(* Logix 5000 AddOnInstructionDefinition export AMCI_SD4840E2_Jog_CCW; software revision 20.03 *)

ADD_ON_INSTRUCTION AMCI_SD4840E2_Jog_CCW   (* revision 1.0, vendor AMCI, ExecuteEnableInFalse *)
VAR_INPUT
   Axis_Status_Bits : INT; {required}
   Programmed_Speed : DINT; {required}
   Acceleration : INT; {required}
   Deceleration : INT; {required}
   Jerk : INT;
END_VAR
VAR_OUTPUT
   EN : BOOL; {access Read Only, visible}
   Jog_CCW_Occurring : BOOL; {access Read Only, visible}
END_VAR
VAR_IN_OUT
   AMCI_SD4840E2_output_data : _000A:SD4840E2_4342D302:O:0; {required}
END_VAR
VAR_OUTPUT
   ER : BOOL; {access Read Only, visible}
END_VAR
VAR
   Upper_Result_X_1000 : DINT;
   command_data_block : INT[10];
        [0]   // Command Bits MSW
        [1]   // Command Bits LSW
        [2]   // Upper Target Position
        [3]   // Lower Target Position
        [4]   // Upper Programmed Speed
        [5]   // Lower Programmed Speed
END_VAR

ROUTINE EnableInFalse   (* ladder *)
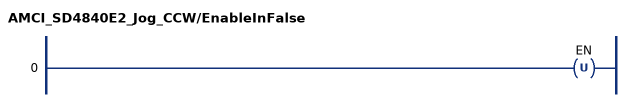
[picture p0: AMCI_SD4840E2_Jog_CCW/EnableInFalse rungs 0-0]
   0: OTU(EN);
END_ROUTINE

ROUTINE Logic   (* ladder *)
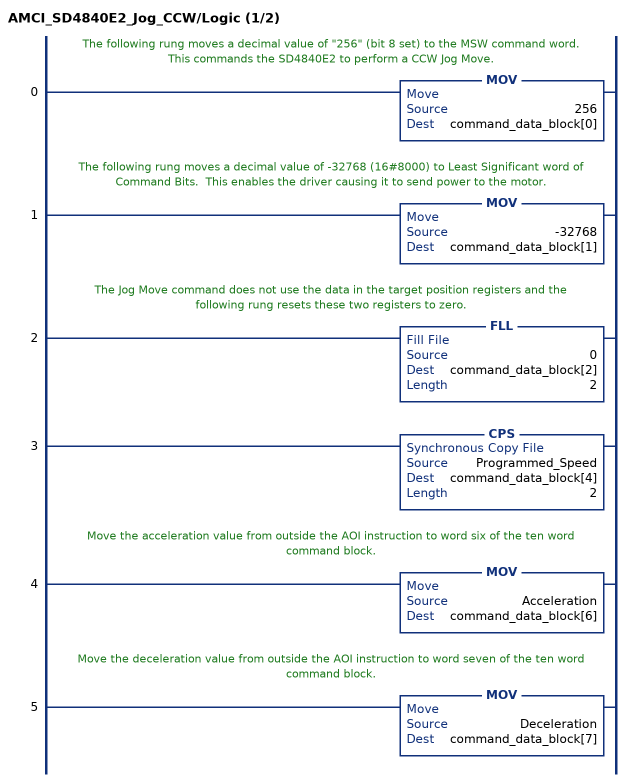
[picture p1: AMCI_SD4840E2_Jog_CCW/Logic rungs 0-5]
   // The following rung moves a decimal value of "256" (bit 8 set) to the MSW command word.  This commands the SD4840E2 to perform a CCW Jog Move.
   0: MOV(256,command_data_block[0]);
   // The following rung moves a decimal value of -32768 (16#8000) to Least Significant word of Command Bits.  This enables the driver causing it to send power to the motor.
   1: MOV(-32768,command_data_block[1]);
   // The Jog Move command does not use the data in the target position registers and the following rung resets these two registers to zero.
   2: FLL(0,command_data_block[2],2);
   3: CPS(Programmed_Speed,command_data_block[4],2);
   // Move the acceleration value from outside the AOI instruction to word six of the ten word command block.
   4: MOV(Acceleration,command_data_block[6]);
   // Move the deceleration value from outside the AOI instruction to word seven of the ten word command block.
   5: MOV(Deceleration,command_data_block[7]);
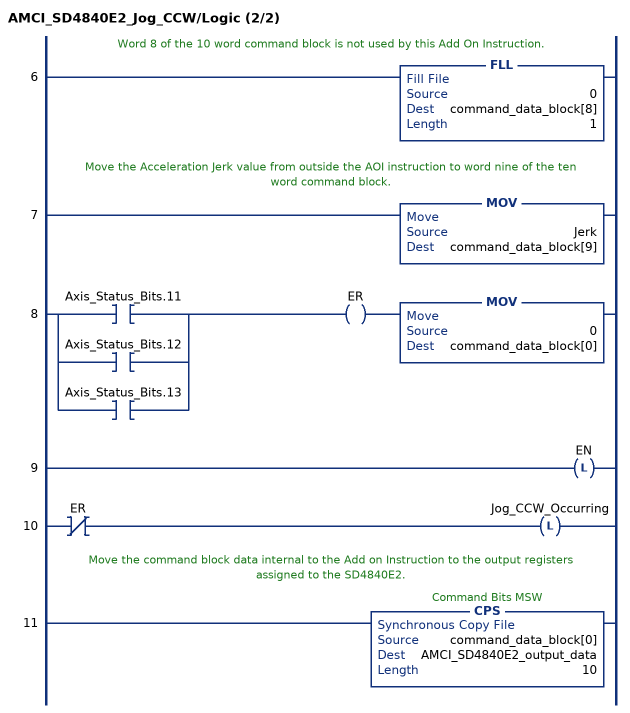
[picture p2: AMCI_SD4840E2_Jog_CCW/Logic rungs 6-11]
   // Word 8 of the 10 word command block is not used by this Add On Instruction.
   6: FLL(0,command_data_block[8],1);
   // Move the Acceleration Jerk value from outside the AOI instruction to word nine of the ten word command block.
   7: MOV(Jerk,command_data_block[9]);
   8: [XIC(Axis_Status_Bits.11) ,XIC(Axis_Status_Bits.12) ,XIC(Axis_Status_Bits.13) ]OTE(ER)MOV(0,command_data_block[0]);
   9: OTL(EN);
   10: XIO(ER)OTL(Jog_CCW_Occurring);
   // Move the command block data internal to the Add on Instruction to the output registers assigned to the SD4840E2.
   11: CPS(command_data_block[0],AMCI_SD4840E2_output_data,10);
END_ROUTINE
END_ADD_ON_INSTRUCTION
